INTERFACE I_TreeNode

METHOD Tick : E_NodeStatus
END_METHOD

METHOD Halt
END_METHOD

METHOD Reset : BOOL
END_METHOD

METHOD GetPath : STRING(255)
END_METHOD

METHOD GetNodeName : STRING(50)
END_METHOD

METHOD SetParent
VAR_INPUT
    ipParent : I_TreeNode;
END_VAR
END_METHOD

METHOD GetProgress : REAL
END_METHOD

METHOD HasError : BOOL
END_METHOD

METHOD GetError : ST_Error
END_METHOD

METHOD ClearError
END_METHOD

END_INTERFACE
